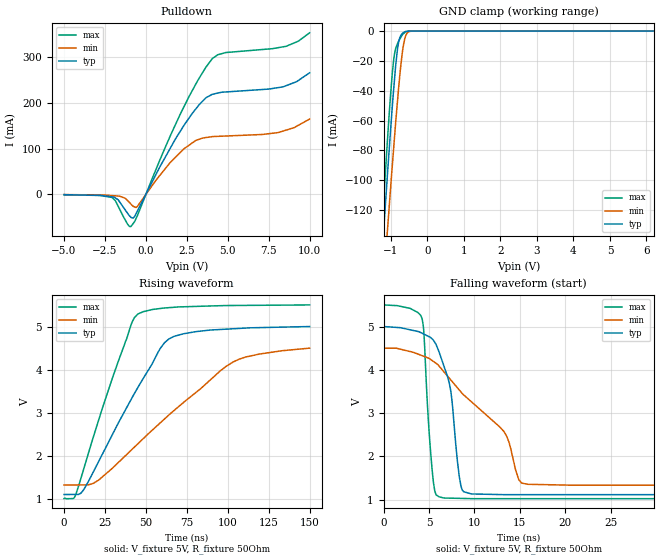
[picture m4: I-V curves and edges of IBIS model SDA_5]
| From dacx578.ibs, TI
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|   SDA Model 5V MODEL
[Model] SDA_5
Model_type   I/O_open_drain
Polarity   Non-Inverting
Enable   Active-Low
Vinl = 1.5
Vinh = 3.5
Vmeas = 2.5
Vref = 2.5
Cref = 15pF
Rref = 50
|   typ   min   max
|   (Nom PVT)   (Fast PVT)  (Slow PVT)
C_comp   2.1240650e-12   1.7782780e-12   2.4710460e-12
|Where nom PVT is Nom process, 5.0V, 27C
|Fast PVT is Strong Process, 5.5V, -40C
|Slow PVT is Weak Process,   4.5V, 125C
[Voltage Range]   5   4.5   5.5
[Temperature Range]   27   125   -40
|Junction temperatures are used for [Temperature Range]
[Pullup Reference]   5   4.5   5.5
[Pulldown Reference]   0   0   0
[Power Clamp Reference]   5   4.5   5.5
[GND Clamp Reference]   0   0   0
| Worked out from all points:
|   slope of the pulldown table from 0 to 0.75 V, typ, clamps not added: 14.1 ohm
|   GND clamp passes 1 mA (typ) near -0.66 V on its own axis
|   falling waveform, V_fixture 5V, R_fixture 50Ohm: 20-80 % time 1.71ns typ, 7.24ns min, 747ps max; typ from 5 V to 1.11 V
|   rising waveform, V_fixture 5V, R_fixture 50Ohm: 20-80 % time 33.6ns typ, 56.1ns min, 23.4ns max; typ from 1.11 V to 5 V
[Pulldown]
|   Voltage   I(typ)   I(min)   I(max)
-5V       -930.5uA   -663.2uA   -951.4uA
-2.077V   -5.548mA   -2.925mA   -6.901mA
-1.7V     -11.88mA   -3.879mA   -25.82mA
-923.8mV  -50.1mA    -21.15mA   -70.87mA
-539.6mV  -38.02mA   -27.46mA   -48.22mA
1.481V    100.6mA    69.56mA    127.6mA
2.341V    152.2mA    100.2mA    193.4mA
3.285V    198mA      121.1mA    256.7mA
4.034V    218.9mA    126.3mA    296.7mA
4.87V     224.3mA    127.7mA    310.7mA
8.354V    235.5mA    138.4mA    323.2mA
9.985V    266.3mA    165mA      354mA
[GND Clamp]
|   Voltage   I(typ)   I(min)   I(max)
-5V       -1.615A    -1.534A    -1.73A
-1.255V   -154.8mA   -188mA     -136.2mA
-1.209V   -137.7mA   -172.3mA   -117.9mA
-1.157V   -118.9mA   -154.7mA   -97.32mA
-1.097V   -96.91mA   -134.3mA   -74.19mA
-955.1mV  -48.75mA   -88.28mA   -26.69mA
-905mV    -33.57mA   -72.52mA   -16.06mA
-828.9mV  -14.06mA   -49.81mA   -9.102mA
-716.4mV  -2.537mA   -20.42mA   -3.774mA
-594.8mV  -291.2uA   -3.235mA   -564.6uA
-390.9mV  -24.42uA   -19.83uA   -42.08uA
9.985V    0A         0A         0A
[POWER Clamp]
|   SCR cell for ESD function. Effects occurr above VDD x 2
|   Voltage   I(typ)   I(min)   I(max)
-5V       0A         0A         0A
0V        0A         0A         0A
10V       0A         0A         0A
[Ramp]
R_load = 50
|   typ   min   max
dV/dt_r   2.3329/3.37194e-008   1.90128/5.58653e-008   2.68877/2.34515e-008
dV/dt_f   2.3329/1.7141e-009   1.90128/7.20754e-009   2.68877/7.43601e-010
[Falling Waveform]
V_fixture = 5V
V_fixture_min = 4.5V
V_fixture_max = 5.5V
R_fixture = 50Ohm
C_fixture = 0F
|   Time   V(typ)   V(min)   V(max)
0s        5V         4.5V       5.5V
4.223ns   4.847V     4.328V     5.196V
5.495ns   4.681V     4.192V     1.389V
6.637ns   4.091V     3.956V     1.035V
7.429ns   3.465V     3.759V     1.031V
8.527ns   1.305V     3.486V     1.025V
9.691ns   1.129V     3.257V     1.02V
13.31ns   1.112V     2.556V     1.019V
15.88ns   1.112V     1.352V     1.019V
150ns     1.112V     1.331V     1.019V
[Rising Waveform]
V_fixture = 5V
V_fixture_min = 4.5V
V_fixture_max = 5.5V
R_fixture = 50Ohm
C_fixture = 0F
|   Time   V(typ)   V(min)   V(max)
0s        1.112V     1.331V     1.019V
7.075ns   1.113V     1.333V     1.098V
11.85ns   1.213V     1.335V     1.678V
20.9ns    1.856V     1.439V     2.802V
41.51ns   3.347V     2.155V     5.095V
44.92ns   3.574V     2.278V     5.282V
59.05ns   4.506V     2.779V     5.419V
67.2ns    4.772V     3.056V     5.445V
106.8ns   4.956V     4.241V     5.488V
150ns     5V         4.5V       5.5V
